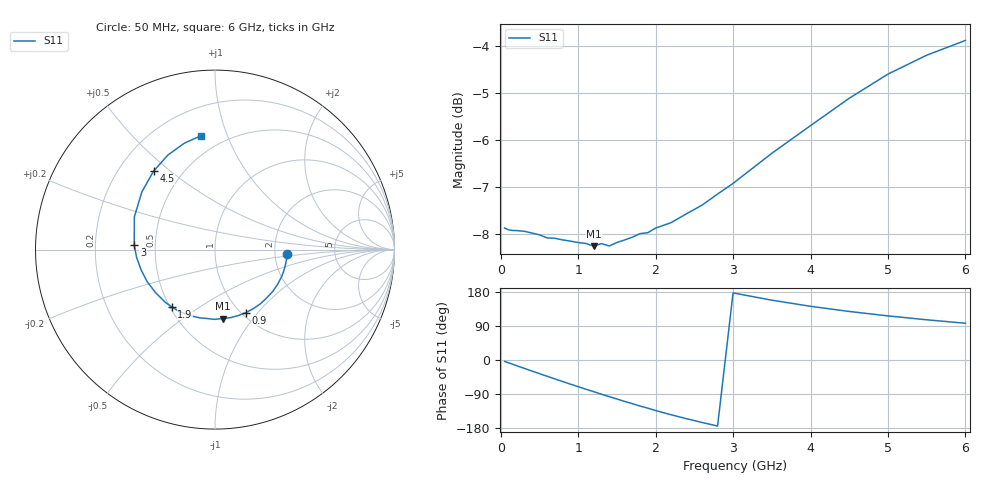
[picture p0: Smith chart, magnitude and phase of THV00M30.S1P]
! SIEMENS Discrete & RF Semiconductors
! BAS70
! Si Schottky Diode in SOT23
! IF = 0.3 mA
! S-Parameters:  February  1997
# GHz  S  MA  R  50
!  f  S11
! GHz  MAG  ANG
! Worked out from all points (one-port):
!   34 points, 50 MHz to 6 GHz, reference 50 ohm
!   lowest |S11| = -8.3 dB at 1.2 GHz (marker M1), VSWR 2.26, Z = 40 - j36.1 ohm
!   |S11| at or under -10 dB: nowhere
!   S11 on the Smith chart (normalised r, x): 50 MHz: 2.34, -0.15; 900 MHz: 1.05, -0.87; 1.9 GHz: 0.51, -0.39; 3 GHz: 0.38, +0.02; 4.5 GHz: 0.35, +0.44; 6 GHz: 0.38, +0.81
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0.05  0.4038 -3.8
0.25  0.4011 -18.2
0.4  0.399 -28.9
0.5  0.3972 -36.0
0.6  0.3942 -43.0
0.7  0.3939 -50.0
0.8  0.3923 -56.8
0.9  0.3911 -63.8
1.1  0.3889 -77.2
1.2  0.3863 -83.6
1.3  0.3888 -90.3
1.4  0.3865 -96.6
1.5  0.3898 -102.9
1.6  0.3922 -109.3
1.8  0.3984 -121.6
1.9  0.3993 -127.2
2  0.4038 -133.4
2.2  0.4092 -144.5
2.4  0.4183 -155.0
2.6  0.4272 -164.9
2.8  0.4389 -174.3
3  0.4505 177.0
3.5  0.485 157.9
4  0.519 141.7
4.5  0.555 128.1
5  0.5888 116.4
5.5  0.6167 106.1
6  0.6394 97.0
